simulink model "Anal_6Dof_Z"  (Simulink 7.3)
settings: Solver=ode45  StartTime=0.0  StopTime=500  RelTol=1e-3
undefined symbols (not defined in the file or in its folder): Acz, Avz, Bcz, Bvz, Ccz, Cvz, Dcz, DiscIntNeverNeededParam, Dvz
libraries: simulink x4

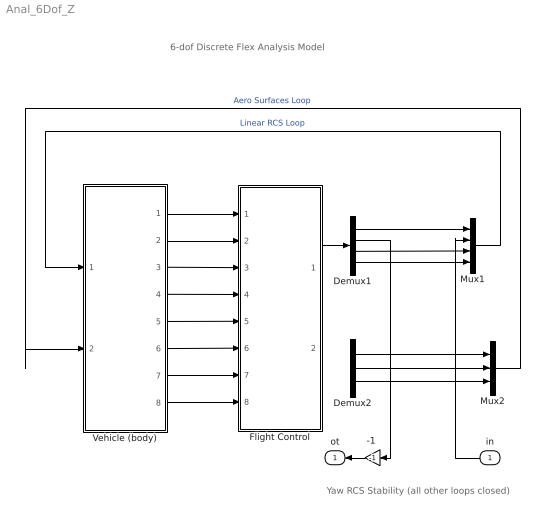
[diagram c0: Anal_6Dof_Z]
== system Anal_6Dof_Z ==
  note: 6-dof Discrete Flex Analysis Model
  note: Yaw RCS Stability (all other loops closed)
  in : Inport  OutDataType=sfix(16)  OutScaling=2^0
  "-1 " : Gain  Gain=-1  ParameterDataType=sfix(16)  ParameterScaling=2^0  OutDataType=sfix(16)  OutScaling=2^0
  Demux1 : Demux
  Demux2 : Demux  Outputs=3
  Flight Control : Subsystem
  Mux1 : Mux
  Mux2 : Mux  Inputs=3
  Vehicle (body) : Subsystem
  ot : Outport  OutDataType=sfix(16)  OutScaling=2^0
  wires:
  Mux2/1 -> Vehicle (body)/2(Aer_pqr)  "Aero Surfaces Loop"
  Mux1/1 -> Vehicle (body)/1(Jet_pqr_Nz)  "Linear RCS Loop"
  "-1 "/1 -> ot/1
  Demux1/4 -> Mux1/4
  Vehicle (body)/1(phi) -> Flight Control/1(phi)
  Vehicle (body)/2(p) -> Flight Control/2(pb)
  Vehicle (body)/3(r) -> Flight Control/3(rb)
  Vehicle (body)/4(bet) -> Flight Control/4(beta)
  Vehicle (body)/5(theta) -> Flight Control/5(thet)
  Vehicle (body)/6(q) -> Flight Control/6(q)
  Vehicle (body)/7(alfa) -> Flight Control/7(alfa)
  Vehicle (body)/8(Nz) -> Flight Control/8(Nz)
  Flight Control/1(Jet_pqr) -> Demux1/1
  Demux2/3 -> Mux2/3
  Demux2/1 -> Mux2/1
  Demux2/2 -> Mux2/2
  Demux1/3 -> Mux1/3
  Demux1/2 -> "-1 "/1
  in/1 -> Mux1/2
  Demux1/1 -> Mux1/1

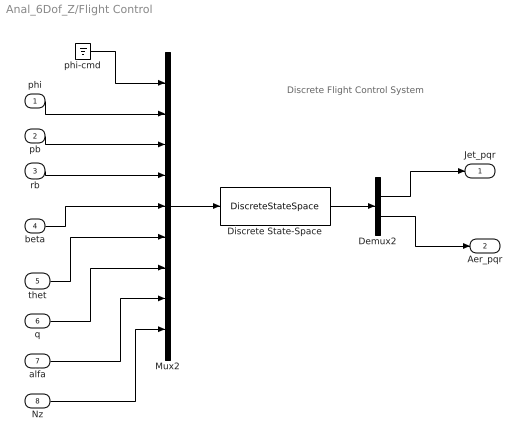
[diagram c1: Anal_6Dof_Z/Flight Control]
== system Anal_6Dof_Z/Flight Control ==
  note: Discrete Flight Control System
  phi : Inport  OutDataType=sfix(16)  OutScaling=2^0
  pb : Inport  Port=2  OutDataType=sfix(16)  OutScaling=2^0
  rb : Inport  Port=3  OutDataType=sfix(16)  OutScaling=2^0
  beta : Inport  Port=4  OutDataType=sfix(16)  OutScaling=2^0
  thet : Inport  Port=5  OutDataType=sfix(16)  OutScaling=2^0
  q : Inport  Port=6  OutDataType=sfix(16)  OutScaling=2^0
  alfa : Inport  Port=7  OutDataType=sfix(16)  OutScaling=2^0
  Nz : Inport  Port=8  OutDataType=sfix(16)  OutScaling=2^0
  Demux2 : Demux  Outputs=[4,3]
  Discrete State-Space : DiscreteStateSpace  A=Acz  B=Bcz  C=Ccz  D=Dcz  SampleTime=0.04
  Mux2 : Mux  Inputs=9
  phi-cmd : Ground
  Jet_pqr : Outport  OutDataType=sfix(16)  OutScaling=2^0
  Aer_pqr : Outport  Port=2  OutDataType=sfix(16)  OutScaling=2^0
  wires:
  Discrete State-Space/1 -> Demux2/1
  Demux2/1 -> Jet_pqr/1
  Demux2/2 -> Aer_pqr/1
  phi/1 -> Mux2/2
  pb/1 -> Mux2/3
  rb/1 -> Mux2/4
  beta/1 -> Mux2/5
  thet/1 -> Mux2/6
  q/1 -> Mux2/7
  Nz/1 -> Mux2/9
  Mux2/1 -> Discrete State-Space/1
  alfa/1 -> Mux2/8
  phi-cmd/1 -> Mux2/1

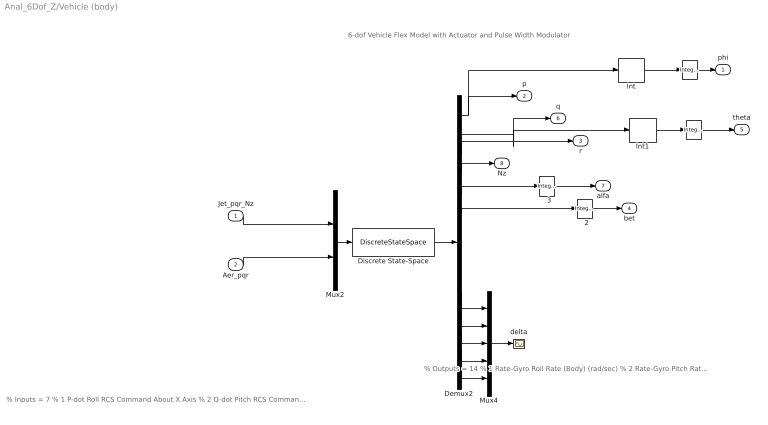
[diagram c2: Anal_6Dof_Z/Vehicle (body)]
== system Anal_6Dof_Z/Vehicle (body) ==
  note: 6-dof Vehicle Flex Model with Actuator and Pulse Width Modulator
  note: % Outputs = 14 % 1 Rate-Gyro Roll Rate (Body) (rad/sec) % 2 Rate-Gyro Pitch Rate (Body) (rad/sec) % 3 Rate-Gyro Yaw Rate (Body) (rad/sec) % 4 Accelerom along Z, (ft/sec^2) Translat. Accelerat. % 5 Angle of attack, alfa, (radians) % 6 Angle of sideslip, beta, (radian) % 7 Change in Altitude, delta-h, (feet) % 8 Forward Acceleration (V-dot) (ft/sec) % 9 Cross Range Velocity (Vcr) (ft/sec) % 10 Left Outboard Deflection (rad) % 11 Left Inboard Deflection (rad) % 12 Right Inboard Deflection (rad) % 13 Right Outboard Deflection (rad) % 14 Rudder Deflection (rad)
  note: % Inputs = 7 % 1 P-dot Roll RCS Command About X Axis % 2 Q-dot Pitch RCS Command About Y Axis % 3 R-dot Yaw RCS Command About Z Axis % 4 Az Normal Acceleration Along Z Axis % 5 P-dot Roll Aero Command About X Axis % 6 Q-dot Pitch Aero Command About Y Axis % 7 R-dot Yaw Aero Command About Z Axis
  Jet_pqr_Nz : Inport  OutDataType=sfix(16)  OutScaling=2^0
  Aer_pqr : Inport  Port=2  OutDataType=sfix(16)  OutScaling=2^0
  "  " : simulink/Discrete/Integer Delay  vinit=0.0  samptime=0.04  NumDelays=1
  "   " : simulink/Discrete/Integer Delay  vinit=0.0  samptime=0.04  NumDelays=1
  "  2" : simulink/Discrete/Integer Delay  vinit=0.0  samptime=0.04  NumDelays=1
  "  3" : simulink/Discrete/Integer Delay  vinit=0.0  samptime=0.04  NumDelays=1
  Demux2 : Demux  Outputs=14
  Discrete State-Space : DiscreteStateSpace  A=Avz  B=Bvz  C=Cvz  D=Dvz  SampleTime=0.04
  Int : DiscreteIntegrator  SampleTime=0.04  OutDataType=sfix(16)  OutScaling=2^0  ICPrevOutput=DiscIntNeverNeededParam  ICPrevScaledInput=DiscIntNeverNeededParam
  Int1 : DiscreteIntegrator  SampleTime=0.04  OutDataType=sfix(16)  OutScaling=2^0  ICPrevOutput=DiscIntNeverNeededParam  ICPrevScaledInput=DiscIntNeverNeededParam
  Mux2 : Mux  Inputs=[4, 3]
  Mux4 : Mux  Inputs=5
  delta : Scope
  phi : Outport  OutDataType=sfix(16)  OutScaling=2^0
  p : Outport  Port=2  OutDataType=sfix(16)  OutScaling=2^0
  r : Outport  Port=3  OutDataType=sfix(16)  OutScaling=2^0
  bet : Outport  Port=4  OutDataType=sfix(16)  OutScaling=2^0
  theta : Outport  Port=5  OutDataType=sfix(16)  OutScaling=2^0
  q : Outport  Port=6  OutDataType=sfix(16)  OutScaling=2^0
  alfa : Outport  Port=7  OutDataType=sfix(16)  OutScaling=2^0
  Nz : Outport  Port=8  OutDataType=sfix(16)  OutScaling=2^0
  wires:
  Mux2/1 -> Discrete State-Space/1
  Demux2/4 -> Nz/1
  Aer_pqr/1 -> Mux2/2
  Jet_pqr_Nz/1 -> Mux2/1
  Demux2/1 -> p/1, Int/1
  Demux2/2 -> q/1, Int1/1
  Demux2/3 -> r/1
  Demux2/14 -> Mux4/5
  Demux2/13 -> Mux4/4
  Demux2/12 -> Mux4/3
  Demux2/11 -> Mux4/2
  Demux2/10 -> Mux4/1
  Demux2/5 -> "  3"/1
  Demux2/6 -> "  2"/1
  Discrete State-Space/1 -> Demux2/1
  Int/1 -> "  "/1
  Int1/1 -> "   "/1
  Mux4/1 -> delta/1
  "  "/1 -> phi/1
  "   "/1 -> theta/1
  "  2"/1 -> bet/1
  "  3"/1 -> alfa/1
